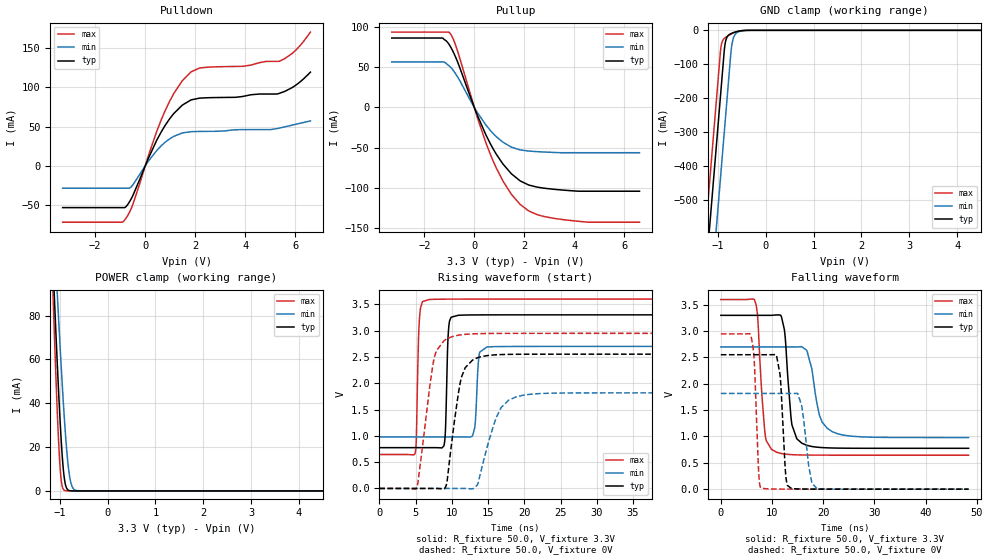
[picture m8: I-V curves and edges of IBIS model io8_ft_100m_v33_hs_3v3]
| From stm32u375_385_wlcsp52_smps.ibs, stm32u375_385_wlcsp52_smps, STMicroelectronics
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[Model]   io8_ft_100m_v33_hs_3v3
Model_type I/O
Polarity   Non-Inverting
Enable   Active-Low
| CAP_THRESHOLD on pad IOFT is "UDTCAPC" :
| Rising=30.0% of vddiom   Falling=70.0% of vddiom
| C_comp min and max val. don't necessarily correlate with the min and max pvt
| but are the smallest and greatest pad capacitance found.
| var   typ   min   max
C_comp   5.13864pF  4.98765pF  5.13964pF
|C_comp_pullup   3.32283pF  3.08588pF  3.41488pF
|C_comp_pulldown   1.81581pF  1.90176pF  1.72476pF
Vinl = 1.35V
Vinh = 1.8V
Vmeas = 1.65V   | Reference voltage for timing measurements
Cref  = 50.0pF   | Timing specification test load capacitance value
Rref  = 1.0MOhm   | Timing specification test load resistance value
Vref  = 1.815V   | Timing specification test load voltage
[Model Spec]
| TIME_THRESHOLD on pin ZIV33M is "CMOS" :
| Rising=50.0% of vddiom   Falling=50.0% of vddiom
Vinl 1.27350V 1.06350V 1.35850V
Vinh 1.78850V 1.51250V 1.89250V
| variable   typ   min   max
[Temperature Range] 25.0 130.0 -40.0
| variable   typ   min   max
[Voltage Range] 3.3V 2.7V 3.6V
| variable   typ   min   max
[POWER Clamp Reference] 3.3V 2.7V 3.6V
| variable   typ   min   max
[GND Clamp Reference] 0V 0V 0V
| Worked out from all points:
|   slope of the pulldown table from 0 to 0.495 V, typ, clamps not added: 14.3 ohm
|   slope of the pullup table from 0 to 0.495 V, typ, clamps not added: 13.8 ohm
|   GND clamp passes 1 mA (typ) near -0.50 V on its own axis
|   POWER clamp passes 1 mA (typ) near -0.85 V on its own axis
|   rising waveform, R_fixture 50.0, V_fixture 3.3V: 20-80 % time 288ps typ, 366ps min, 294ps max; typ from 0.776 V to 3.3 V
|   falling waveform, R_fixture 50.0, V_fixture 3.3V: 20-80 % time 1.16ns typ, 2.01ns min, 1.11ns max; typ from 3.3 V to 0.776 V
|   rising waveform, R_fixture 50.0, V_fixture 0V: 20-80 % time 1.54ns typ, 2.42ns min, 1.63ns max; typ from 0 V to 2.55 V
|   falling waveform, R_fixture 50.0, V_fixture 0V: 20-80 % time 828ps typ, 1.33ns min, 709ps max; typ from 2.55 V to 0 V
[POWER Clamp]
-3.3V     1.376A     1.183A     1.687A
-1.15V    107mA      132mA      94.23mA
-1.14V    101.7mA    127.5mA    87.74mA
-1.11V    86.11mA    114.3mA    68.77mA
-1.05V    56.42mA    88.49mA    34.19mA
-1V       34.12mA    67.92mA    12.34mA
-960mV    19.14mA    52.36mA    3.231mA
-900mV    4.863mA    31.3mA     221.9uA
-840mV    665uA      14.67mA    12.78uA
-790mV    105.7uA    5.908mA    1.173uA
-650mV    562.2nA    165.6uA    2.035nA
6.6V      0A         0A         0A
[GND Clamp]
-3.3V     -4.192A    -4.434A    -4.059A
-1.25V    -707.2mA   -948.8mA   -574.2mA
-950mV    -197.2mA   -438.8mA   -64.18mA
-940mV    -180.2mA   -421.8mA   -51.24mA
-870mV    -61.19mA   -302.8mA   -24.27mA
-850mV    -38.62mA   -268.8mA   -21.84mA
-800mV    -17.58mA   -183.8mA   -16.98mA
-730mV    -9.777mA   -65.72mA   -11.28mA
-710mV    -8.51mA    -43.04mA   -9.847mA
-620mV    -4.247mA   -8.765mA   -4.565mA
-390mV    -85.77uA   -309.6uA   -31.83uA
6.6V      2.503nA    356.6nA    1.779nA
| variable   typ   min   max
[Pullup Reference] 3.3V 2.7V 3.6V
| variable   typ   min   max
[Pulldown Reference] 0V 0V 0V
[Pullup]
-3.3V     86.14mA    56.49mA    93.49mA
-1.28V    86.12mA    56.49mA    93.49mA
-960mV    75.73mA    50.26mA    91.62mA
-710mV    59.63mA    39.99mA    73.75mA
120mV     -9.578mA   -6.208mA   -12.33mA
650mV     -45.52mA   -28.81mA   -58.82mA
1.14V     -69.93mA   -42.96mA   -90.97mA
1.83V     -90.96mA   -52.61mA   -120.1mA
2.51V     -98.71mA   -54.73mA   -132.8mA
3.3V      -101.8mA   -55.87mA   -138mA
4.55V     -103.8mA   -56.04mA   -142.2mA
6.6V      -103.8mA   -56.04mA   -142.2mA
[Pulldown]
-3.3V     -53.27mA   -28.52mA   -71.84mA
-850mV    -53.27mA   -28.52mA   -70.02mA
-500mV    -38.18mA   -24.47mA   -49.51mA
460mV     32.61mA    19.53mA    43.99mA
800mV     51.7mA     30.09mA    70.55mA
1.14V     66.56mA    37.47mA    92mA
1.48V     77.24mA    41.82mA    108.3mA
1.83V     83.91mA    43.43mA    119.6mA
2.17V     86.16mA    43.73mA    124.5mA
5.35V     92.17mA    47.94mA    133mA
5.95V     101.3mA    52.36mA    145.4mA
6.6V      119.3mA    57.17mA    170.3mA
[Ramp]
dV/dt_r 1.53142V/1.54534ns 1.09016V/2.38307ns 1.76896V/1.62888ns
dV/dt_f 1.51461V/1.15883ns 1.03187V/1.87538ns 1.77292V/1.10783ns
R_load = 50.0
| Removed startup time: 0s 0s 0s  .
| Removed end time: 48.4ns.
[Rising Waveform]
R_fixture   = 50.0
V_fixture   = 3.3V
V_fixture_min = 2.7V
V_fixture_max = 3.6V
0s        775.7mV    980.2mV    645.1mV
4.95ns    775.7mV    980.2mV    678.6mV
5.45ns    775.7mV    980.2mV    3.023V
5.95ns    775.7mV    980.2mV    3.551V
8.95ns    838.1mV    980.2mV    3.598V
9.9ns     3.255V     980.2mV    3.599V
12.85ns   3.298V     997.7mV    3.6V
13.75ns   3.299V     2.519V     3.6V
14.85ns   3.3V       2.69V      3.6V
48.4ns    3.3V       2.7V       3.6V
| Removed startup time: 0s 0s 0s  .
| Removed end time: 48.4ns.
[Falling Waveform]
R_fixture   = 50.0
V_fixture   = 3.3V
V_fixture_min = 2.7V
V_fixture_max = 3.6V
0s        3.3V       2.7V       3.6V
6.55ns    3.3V       2.7V       3.601V
7.2ns     3.3V       2.7V       3.264V
8.6ns     3.3V       2.7V       1.092V
9.9ns     3.3V       2.7V       755.7mV
11.85ns   3.271V     2.7V       676.5mV
13.9ns    1.217V     2.7V       655mV
15.8ns    874.6mV    2.706V     649.1mV
21.75ns   781.6mV    1.092V     645.5mV
48.4ns    775.7mV    980.2mV    645.1mV
| Removed startup time: 0s 0s 0s  .
| Removed end time: 48.4ns.
[Rising Waveform]
R_fixture   = 50.0
V_fixture   = 0V
V_fixture_min = 0V
V_fixture_max = 0V
0s        11.93nV    102.1nV    24.43nV
5.15ns    10.62nV    101.6nV    12.19mV
7.55ns    8.28uV     100.7nV    2.466V
9.15ns    33.61mV    126.1nV    2.83V
9.75ns    614.1mV    290nV      2.871V
11.35ns   2.124V     3.868uV    2.922V
13.5ns    2.482V     62.15mV    2.942V
16.15ns   2.541V     1.353V     2.947V
18.8ns    2.55V      1.737V     2.948V
48.4ns    2.552V     1.817V     2.948V
| Removed startup time: 0s 0s 0s  .
| Removed end time: 48.4ns.
[Falling Waveform]
R_fixture   = 50.0
V_fixture   = 0V
V_fixture_min = 0V
V_fixture_max = 0V
0s        2.552V     1.817V     2.948V
5.95ns    2.552V     1.817V     2.879V
7.9ns     2.552V     1.817V     18.03mV
10.9ns    2.526V     1.817V     2.191mV
11.65ns   2.084V     1.817V     1.556mV
12.75ns   205.3mV    1.817V     953uV
13.85ns   9.376mV    1.817V     597uV
15.8ns    3.386mV    1.586V     272.1uV
18.8ns    899.3uV    9.201mV    84.99uV
48.4ns    95.25nV    2.302uV    44.87nV
